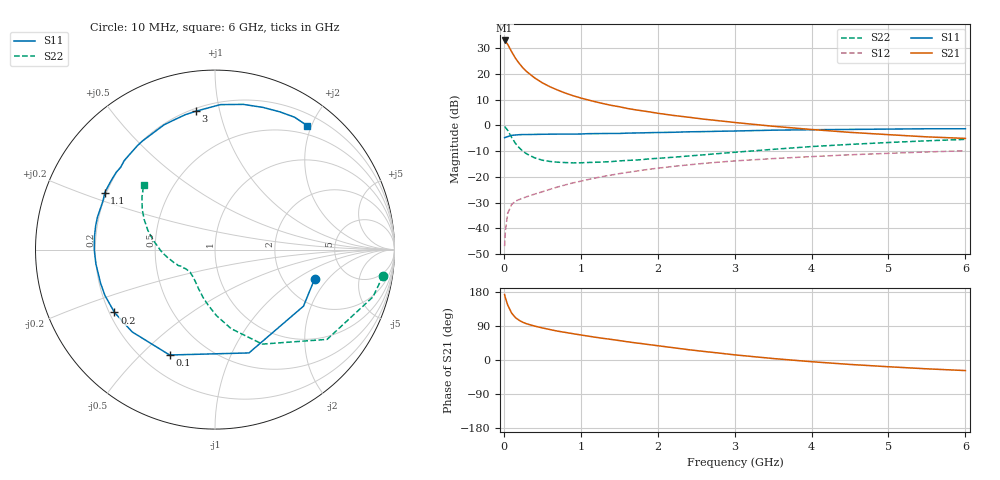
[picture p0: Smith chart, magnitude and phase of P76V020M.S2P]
! SIEMENS Small Signal Semiconductors
! BFP196
! Si NPN RF Bipolar Junction Transistor in SOT143
! VCE = 6 V  IC = 20 mA
! Common Emitter S-Parameters:  May  1996
# GHz  S  MA  R  50
!  f  S11  S21  S12  S22
! GHz  MAG  ANG  MAG  ANG  MAG  ANG  MAG  ANG
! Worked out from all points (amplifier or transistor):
!   36 points, 10 MHz to 6 GHz, reference 50 ohm
!   highest |S21| = 33.0 dB at 10 MHz (marker M1)
!   |S21| within 3 dB of that: start of sweep to 76.62 MHz
!   unconditionally stable (mu >= 1): 716.2 MHz to 3.423 GHz
!   at 250 MHz: K = 0.58, MSG = 25.3 dB, |S12| = -28.2 dB
!   at 1.4 GHz: K = 1.11, MAG = 11.5 dB, |S12| = -19.3 dB
!   at 6 GHz: K = 0.96, MSG = 2.4 dB, |S12| = -9.8 dB
!   S11 on the Smith chart (normalised r, x): 10 MHz: 2.95, -1.46; 100 MHz: 0.31, -0.61; 200 MHz: 0.22, -0.27; 1.1 GHz: 0.19, +0.23; 3 GHz: 0.22, +0.85; 6 GHz: 0.36, +1.94
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0.01  0.5785 -16.5  44.77 172.6  0.0045 82.4  0.9479 -8.8
0.02  0.5851 -32.6  43.33 164.1  0.0088 78.4  0.9184 -16.7
0.05  0.606 -71.8  37.59 145.1  0.0195 61.7  0.8001 -38.7
0.1  0.6394 -113.3  27.28 124.2  0.0289 47.4  0.5888 -63.4
0.15  0.6507 -135.2  20.31 112.0  0.0337 42.5  0.45 -78.4
0.2  0.6604 -148.0  15.99 104.6  0.0363 40.5  0.3675 -88.8
0.25  0.6644 -157.4  13.02 99.2  0.0387 41.0  0.3123 -96.9
0.3  0.6644 -163.7  11.01 95.3  0.0413 42.0  0.2783 -103.3
0.4  0.6683 -173.2  8.389 89.5  0.0462 44.6  0.2344 -113.4
0.5  0.6729 -180.0  6.729 84.7  0.0514 47.0  0.2109 -120.7
0.6  0.6753 174.1  5.635 80.3  0.0573 48.9  0.1993 -126.4
0.8  0.6795 164.7  4.246 72.8  0.0698 51.1  0.1897 -134.8
0.9  0.6782 160.5  3.777 69.4  0.0764 51.9  0.1868 -137.9
1.1  0.6914 152.8  3.111 62.9  0.0891 52.1  0.1904 -142.4
1.3  0.6958 145.1  2.638 56.9  0.1025 51.5  0.1949 -146.8
1.6  0.7082 135.6  2.144 48.3  0.1219 49.6  0.2087 -152.2
2.2  0.7352 118.1  1.565 32.5  0.1597 43.8  0.2407 -162.7
3  0.7782 97.9  1.141 13.6  0.2042 34.2  0.3006 -178.4
3.5  0.8082 87.9  0.963 3.9  0.2267 28.0  0.3429 172.3
4.5  0.836 71.4  0.733 -11.7  0.2686 16.9  0.428 157.1
5.5  0.8606 59.0  0.599 -23.3  0.3049 6.2  0.5021 144.1
6  0.8607 53.3  0.559 -27.9  0.322 0.4  0.5353 138.0
